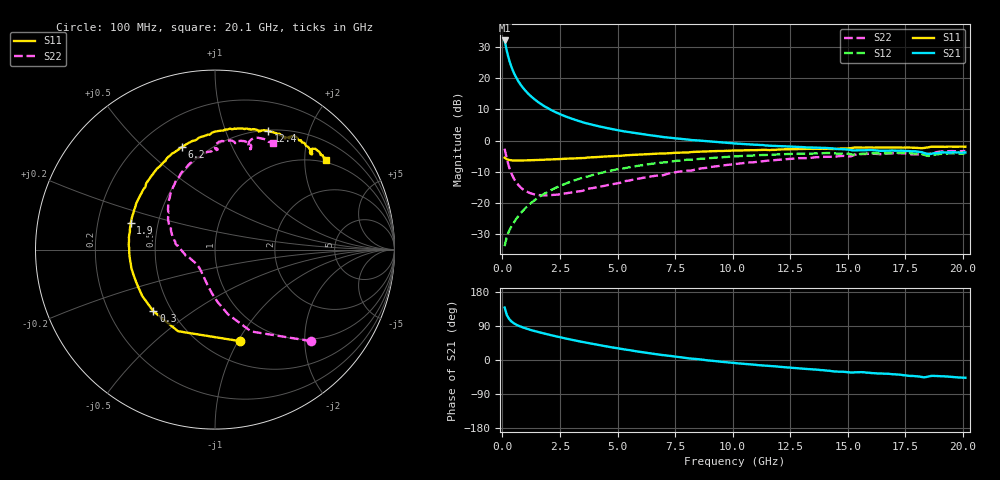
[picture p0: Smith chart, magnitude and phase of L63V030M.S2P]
!  Infineon Technologies AG
! BFR380L3 , PF131585-7, No.6, Th 09.10.01, soldered on pcb-board, measured with PP GSG850
!  Vce=3.0 V,  Ic=30.0 mA
! Common Emitter S-Parameters:  15. November 2001
#  GHz  S  MA  R  50
! f  S11  S21  S12  S22
! GHz  Mag  Ang  Mag  Ang  Mag  Ang  Mag  Ang
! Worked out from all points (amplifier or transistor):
!   201 points, 100 MHz to 20.1 GHz, reference 50 ohm
!   highest |S21| = 32.2 dB at 100 MHz (marker M1)
!   |S21| within 3 dB of that: start of sweep to 184.4 MHz
!   unconditionally stable (mu >= 1): 1.229 GHz to 4.298 GHz
!   at 3.4 GHz: K = 1.02, MAG = 8.3 dB, |S12| = -12.2 dB
!   at 10.1 GHz: K = 0.96, MSG = 2.1 dB, |S12| = -5.1 dB
!   at 20.1 GHz: K = 0.98, MSG = 0.1 dB, |S12| = -4.1 dB
!   S11 on the Smith chart (normalised r, x): 100 MHz: 0.72, -1.02; 300 MHz: 0.40, -0.36; 1.9 GHz: 0.35, +0.14; 6.2 GHz: 0.37, +0.66; 12.4 GHz: 0.51, +1.42; 20.1 GHz: 0.94, +2.54
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0.1  0.5297 -74.5  40.76 138.5  0.01993 62.4  0.7385 -43.6
0.2  0.4991 -114.4  27.07 118.0  0.02879 56.9  0.4987 -66.2
0.3  0.4857 -135.0  19.55 107.8  0.03544 57.3  0.3676 -78.6
0.4  0.4808 -147.5  15.16 101.5  0.04162 58.8  0.2921 -87.2
0.5  0.4755 -156.0  12.33 96.9  0.04778 60.9  0.2451 -93.9
0.6  0.4753 -162.2  10.37 93.5  0.05452 62.6  0.2135 -99.4
0.7  0.4772 -167.3  8.964 90.5  0.06096 63.8  0.1914 -104.3
0.8  0.4762 -171.2  7.879 88.0  0.06784 64.8  0.1753 -108.7
1  0.4782 -177.9  6.355 83.7  0.08156 65.9  0.1543 -116.3
1.2  0.4816 176.7  5.327 79.8  0.09532 66.4  0.1427 -122.8
1.5  0.4851 169.9  4.298 74.7  0.1164 66.2  0.1337 -131.0
1.9  0.4928 162.3  3.434 68.6  0.1442 64.9  0.1309 -140.2
2.6  0.5052 151.1  2.563 58.8  0.1925 61.5  0.1382 -153.1
3.5  0.5221 138.0  1.961 47.3  0.2527 55.8  0.1556 -165.2
4.8  0.5594 122.5  1.517 32.9  0.3322 47.1  0.199 176.8
6.2  0.6007 108.0  1.248 19.4  0.4085 37.2  0.2545 160.6
6.8  0.616 102.5  1.165 14.2  0.4371 32.8  0.2742 153.7
10.1  0.6891 78.2  0.8967 -7.9  0.5544 11.3  0.4183 124.1
12.4  0.7231 65.9  0.8066 -19.7  0.6072 -2.8  0.5028 105.3
13.5  0.732 60.7  0.7726 -24.7  0.619 -9.2  0.5306 97.9
16.8  0.7716 48.2  0.6903 -36.5  0.6256 -25.0  0.6197 77.5
20.1  0.7949 38.7  0.6412 -46.9  0.6204 -38.6  0.6766 61.6
